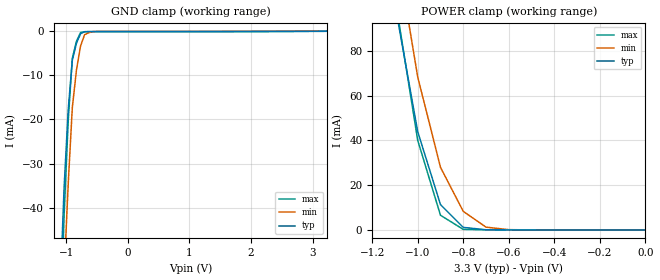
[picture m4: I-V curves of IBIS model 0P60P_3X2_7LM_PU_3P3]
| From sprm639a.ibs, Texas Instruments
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|   Model Cell 0P60P_3X2_7LM_PU_3P3
|IQ0442FS_40P60P_3X2_PU_3P3
[Model]   0P60P_3X2_7LM_PU_3P3
Model_type   Input
Polarity   Non-Inverting
Vinl =  1.55
Vinh =  1.75
C_comp   1.2p   1.2p   1.2p
[Model Spec]
Vinl   1.55   1.42   1.68
Vinh   1.75   1.55   1.85
[Temperature Range]   25   155   -40
[Voltage Range]   3.3   2.97   3.63
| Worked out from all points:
|   GND clamp passes 1 mA (typ) near -0.78 V on its own axis
|   POWER clamp passes 1 mA (typ) near -0.79 V on its own axis
[POWER_clamp]
|   voltage   I(typ)   I(min)   I(max)
-3.3V     1.823A     2.351A     1.96A
-1.1V     100.7mA    129.7mA    104mA
-1.067V   81.78mA    109.2mA    82.67mA
-1.033V   62.85mA    88.78mA    61.35mA
-1V       43.91mA    68.32mA    40.03mA
-900mV    11.33mA    27.98mA    6.575mA
-800mV    1.159mA    8.31mA     262.7uA
-700mV    89.5uA     1.262mA    78.79uA
-600mV    47.29uA    138.9uA    65.15uA
0V        173.5pA    245.5pA    190.9pA
[GND_clamp]
|   voltage   I(typ)   I(min)   I(max)
-3.3V     -1.38A     -1.323A    -2.074A
-1.1V     -59.6mA    -79.12mA   -70.72mA
-1.033V   -35.5mA    -55.25mA   -41.84mA
-966.7mV  -17.83mA   -34.66mA   -20.32mA
-900mV    -6.605mA   -17.33mA   -6.158mA
-833.3mV  -2.754mA   -8.869mA   -2.319mA
-766.7mV  -592uA     -3.357mA   -314.7uA
-700mV    -119.5uA   -797.1uA   -143.3uA
-566.7mV  -87.28uA   -106.7uA   -139uA
3.233V    -4.592uA   11.77uA    -37.4uA
